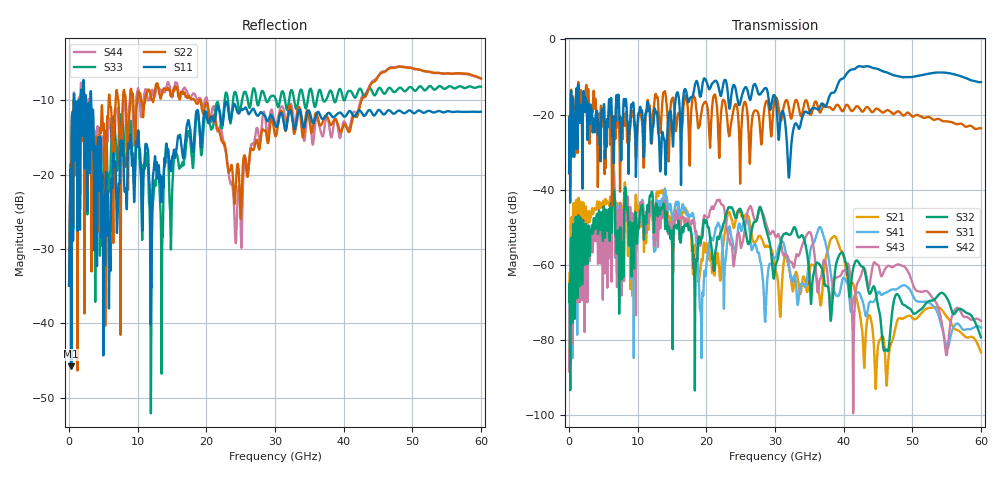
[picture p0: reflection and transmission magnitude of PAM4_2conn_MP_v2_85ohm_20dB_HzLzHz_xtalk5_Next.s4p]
! Info: Touchstone file created by Circ.  Input file=FAB50GbE_2conn_Midplane_Examax_Topo2_v2_85ohm_20dB_HzLzHz.circ
# Hz S RI R 50
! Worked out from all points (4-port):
!   6000 points, 10 MHz to 60 GHz, reference 50 ohm
!   strongest paths, dB at 10 MHz, 15.01 GHz, 30.01 GHz, 45.01 GHz, 60 GHz:
!     S42: -35.5, -24.0, -15.3, -7.9, -11.4
!     S31: -35.7, -15.8, -15.8, -18.5, -23.7
!     S32: -69.9, -54.7, -61.2, -71.0, -79.3
!     S43: -88.4, -53.3, -52.2, -60.1, -75.0
!     S41: -88.1, -47.1, -58.1, -67.4, -76.7
!     S21: -69.5, -50.8, -60.8, -81.7, -83.3
!   lowest |S11| = -45.8 dB at 320 MHz (marker M1), VSWR 1.01, Z = 50.1 + j0.51 ohm
!   |S11| at or under -10 dB: start of sweep to 683.6 MHz; 2.465 GHz to 3.106 GHz (640.9 MHz wide, 23 % of centre); 3.226 GHz to end of sweep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
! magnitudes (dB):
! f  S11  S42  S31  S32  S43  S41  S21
! 10 MHz  -34.9  -35.5  -35.7  -69.9  -88.4  -88.1  -69.5
! 320 MHz  -45.8  -14.1  -13.6  -52.9  -59.8  -54.2  -47.7
! 14.02 GHz  -18.4  -32.9  -14.1  -50.5  -44.4  -40.2  -43.2
! 19.27 GHz  -16.0  -14.4  -19.8  -52.8  -53.0  -79.3  -59.1
! 21.74 GHz  -10.8  -12.3  -24.9  -52.9  -42.9  -48.8  -58.3
! 32.06 GHz  -11.6  -36.5  -18.6  -52.0  -58.9  -60.5  -60.9
! 60 GHz  -11.5  -11.4  -23.7  -79.3  -75.0  -76.7  -83.3
